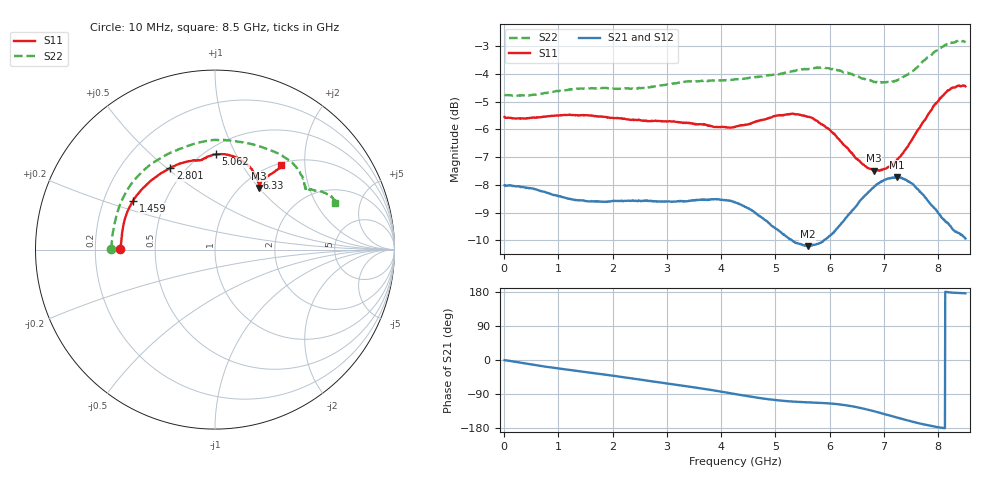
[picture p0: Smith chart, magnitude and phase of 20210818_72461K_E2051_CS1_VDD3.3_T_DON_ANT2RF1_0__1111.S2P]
!Agilent Technologies,E5071C,MY46417908,A.11.23
!Date: Wed Aug 18 14:24:52 2021
!Data & Calibration Information:
!Freq	S11:SOLT2(ON)	S21:SOLT2(ON)	S12:SOLT2(ON)	S22:SOLT2(ON)
!PortZ  Port1:50+j0  Port2:50+j0
!Above PortZ is port z conversion or system Z0 setting when saving the data.
!When reading, reference impedance value at option line is always used.
# Hz S dB R 50
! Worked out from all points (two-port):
!   1601 points, 10 MHz to 8.5 GHz, reference 50 ohm
!   highest |S21| = -7.72 dB at 7.242 GHz (marker M1); lowest = -10.2 dB at 5.597 GHz (marker M2)
!   |S21| within 3 dB of the highest: start of sweep to end of sweep
!   lowest |S11| = -7.5 dB at 6.813 GHz (marker M3), VSWR 2.46, Z = 59.8 + j50 ohm
!   |S11| at or under -10 dB: nowhere
!   |S22| runs from -4.8 to -2.8 dB; largest |S21 - S12| = 0.0018
!   S11 on the Smith chart (normalised r, x): 10 MHz: 0.31, +0.00; 1.459 GHz: 0.33, +0.25; 2.801 GHz: 0.41, +0.52; 5.062 GHz: 0.56, +0.83; 6.33 GHz: 1.05, +1.07; 8.5 GHz: 1.04, +1.52
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1e7  -5.56 179.7  -8.01 -0.4  -8.01 -0.3  -4.75 179.6
7.847125e8  -5.54 164.2  -8.28 -18.2  -8.28 -18.2  -4.69 158.0
1.426769e9  -5.49 149.8  -8.56 -30.6  -8.56 -30.5  -4.53 139.1
1.458606e9  -5.49 149.1  -8.56 -31.2  -8.57 -31.1  -4.53 138.2
2.1325e9  -5.60 133.3  -8.58 -44.0  -8.59 -44.1  -4.54 118.6
2.801088e9  -5.69 118.6  -8.59 -57.8  -8.59 -57.9  -4.45 102.3
2.843538e9  -5.70 117.7  -8.60 -58.7  -8.59 -58.8  -4.43 101.4
3.607638e9  -5.82 104.2  -8.54 -74.5  -8.53 -74.5  -4.27 86.6
4.255e9  -5.91 98.1  -8.63 -89.9  -8.62 -89.9  -4.20 76.4
4.727256e9  -5.67 94.3  -9.15 -100.7  -9.15 -100.7  -4.10 69.3
5.06155e9  -5.50 89.5  -9.65 -106.6  -9.66 -106.5  -4.01 63.4
5.597481e9  -5.56 77.6  -10.21 -111.7  -10.23 -111.7  -3.84 53.3
5.671769e9  -5.59 75.9  -10.18 -112.2  -10.20 -112.1  -3.81 51.8
5.979531e9  -5.98 67.7  -9.87 -114.4  -9.90 -114.4  -3.80 46.1
6.329744e9  -6.68 59.7  -9.11 -120.2  -9.13 -120.4  -3.96 39.8
6.812612e9  -7.49 54.4  -8.09 -135.0  -8.09 -135.0  -4.30 34.8
7.088538e9  -7.35 54.9  -7.77 -145.8  -7.78 -145.8  -4.30 33.4
7.242419e9  -7.09 55.4  -7.72 -151.8  -7.73 -151.8  -4.23 32.7
7.539569e9  -6.30 54.7  -7.99 -163.3  -7.99 -163.3  -3.89 31.4
7.916312e9  -5.16 52.4  -8.82 -175.2  -8.80 -175.3  -3.23 27.2
8.171012e9  -4.62 51.5  -9.37 179.2  -9.35 179.2  -2.94 24.4
8.5e9  -4.45 51.8  -9.93 176.1  -9.89 176.0  -2.87 21.2
